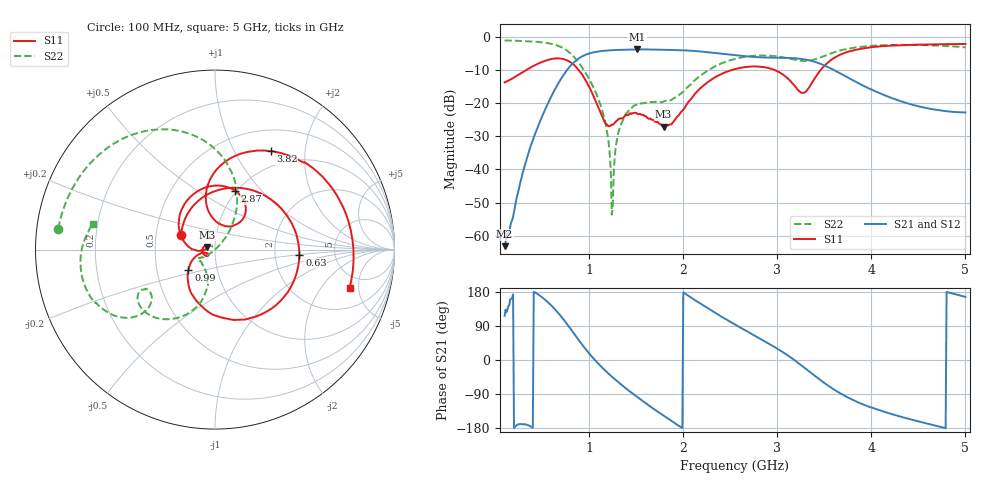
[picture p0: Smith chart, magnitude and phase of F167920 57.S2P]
!  2-Port S-parameters saved by WinCal
! VAR MeasName=S-Parameters (CALIBRATED_DATA) read from VNA (N5242A)
! VAR MeasDate=2016-11-22 9:58:21
! VAR NAME=F167920 57
! VAR FILENAME=F167920 57.S2P
! VAR DATE=2016-11-22 9:58:21
! VAR PHYS_PORTS=1,2
# Hz S DB R 50
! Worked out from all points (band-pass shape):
!   491 points, 100 MHz to 5 GHz, reference 50 ohm
!   highest |S21| = -3.79 dB at 1.51 GHz (marker M1); lowest = -63.2 dB at 100 MHz (marker M2)
!   |S21| within 3 dB of the highest: 875.2 MHz to 3.284 GHz (2.409 GHz wide, 116 % of centre)
!   lowest |S11| = -27.1 dB at 1.79 GHz (marker M3), VSWR 1.09, Z = 45.9 + j1.3 ohm
!   |S11| at or under -10 dB: start of sweep to 330.3 MHz; 885.9 MHz to 2.518 GHz (1.632 GHz wide, 95.9 % of centre); 2.969 GHz to 3.461 GHz (492.1 MHz wide, 15.3 % of centre)
!   |S22| runs from -53.6 to -1.1 dB; largest |S21 - S12| = 0.0017
!   S11 on the Smith chart (normalised r, x): 100 MHz: 0.67, +0.11; 630 MHz: 2.76, -0.20; 990 MHz: 0.73, -0.17; 2.87 GHz: 0.98, +0.73; 3.82 GHz: 0.78, +1.41; 5 GHz: 3.66, -3.94
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1e8  -13.76 157.2  -63.16 116.5  -63.38 114.1  -1.10 172.4
4.2e8  -8.60 67.5  -29.62 178.7  -29.63 178.6  -1.45 145.6
6.3e8  -6.54 -3.4  -16.14 135.3  -16.14 135.4  -2.35 119.8
7.8e8  -7.33 -62.3  -9.45 89.5  -9.45 89.6  -4.50 94.0
9.2e8  -11.17 -118.9  -5.93 42.1  -5.92 42.2  -9.06 70.0
9.9e8  -14.62 -142.9  -5.11 19.9  -5.11 20.0  -12.25 61.2
1.17e9  -26.00 -158.9  -4.19 -28.0  -4.19 -28.0  -25.70 45.9
1.2e9  -26.87 -152.1  -4.11 -35.0  -4.11 -35.0  -30.46 44.7
1.24e9  -26.47 -142.1  -4.04 -43.8  -4.04 -43.8  -53.65 51.7
1.26e9  -26.34 -139.0  -4.02 -48.3  -4.02 -48.3  -41.53 -135.5
1.32e9  -24.66 -144.0  -3.93 -60.8  -3.92 -60.8  -27.85 -144.1
1.51e9  -23.16 179.5  -3.79 -97.6  -3.79 -97.6  -20.52 -152.0
1.74e9  -26.08 154.9  -3.87 -138.3  -3.87 -138.3  -19.67 -141.9
1.79e9  -27.06 161.4  -3.91 -147.0  -3.91 -147.0  -19.53 -134.5
2.1e9  -18.09 179.6  -4.20 162.0  -4.20 161.9  -13.71 -101.3
2.55e9  -9.74 114.2  -5.55 93.7  -5.57 93.6  -6.67 -123.4
2.87e9  -9.21 71.0  -6.24 48.9  -6.26 49.0  -5.63 -142.7
3.26e9  -16.91 67.3  -6.69 -15.0  -6.69 -15.0  -7.25 -148.6
3.37e9  -13.81 98.5  -7.30 -36.1  -7.31 -36.0  -7.04 -142.3
3.82e9  -4.01 60.6  -13.36 -107.3  -13.39 -107.1  -3.27 -148.8
4.19e9  -2.70 29.5  -18.19 -140.7  -18.22 -140.3  -2.49 -163.4
5e9  -2.17 -15.8  -22.82 166.7  -22.82 167.0  -3.17 168.2
